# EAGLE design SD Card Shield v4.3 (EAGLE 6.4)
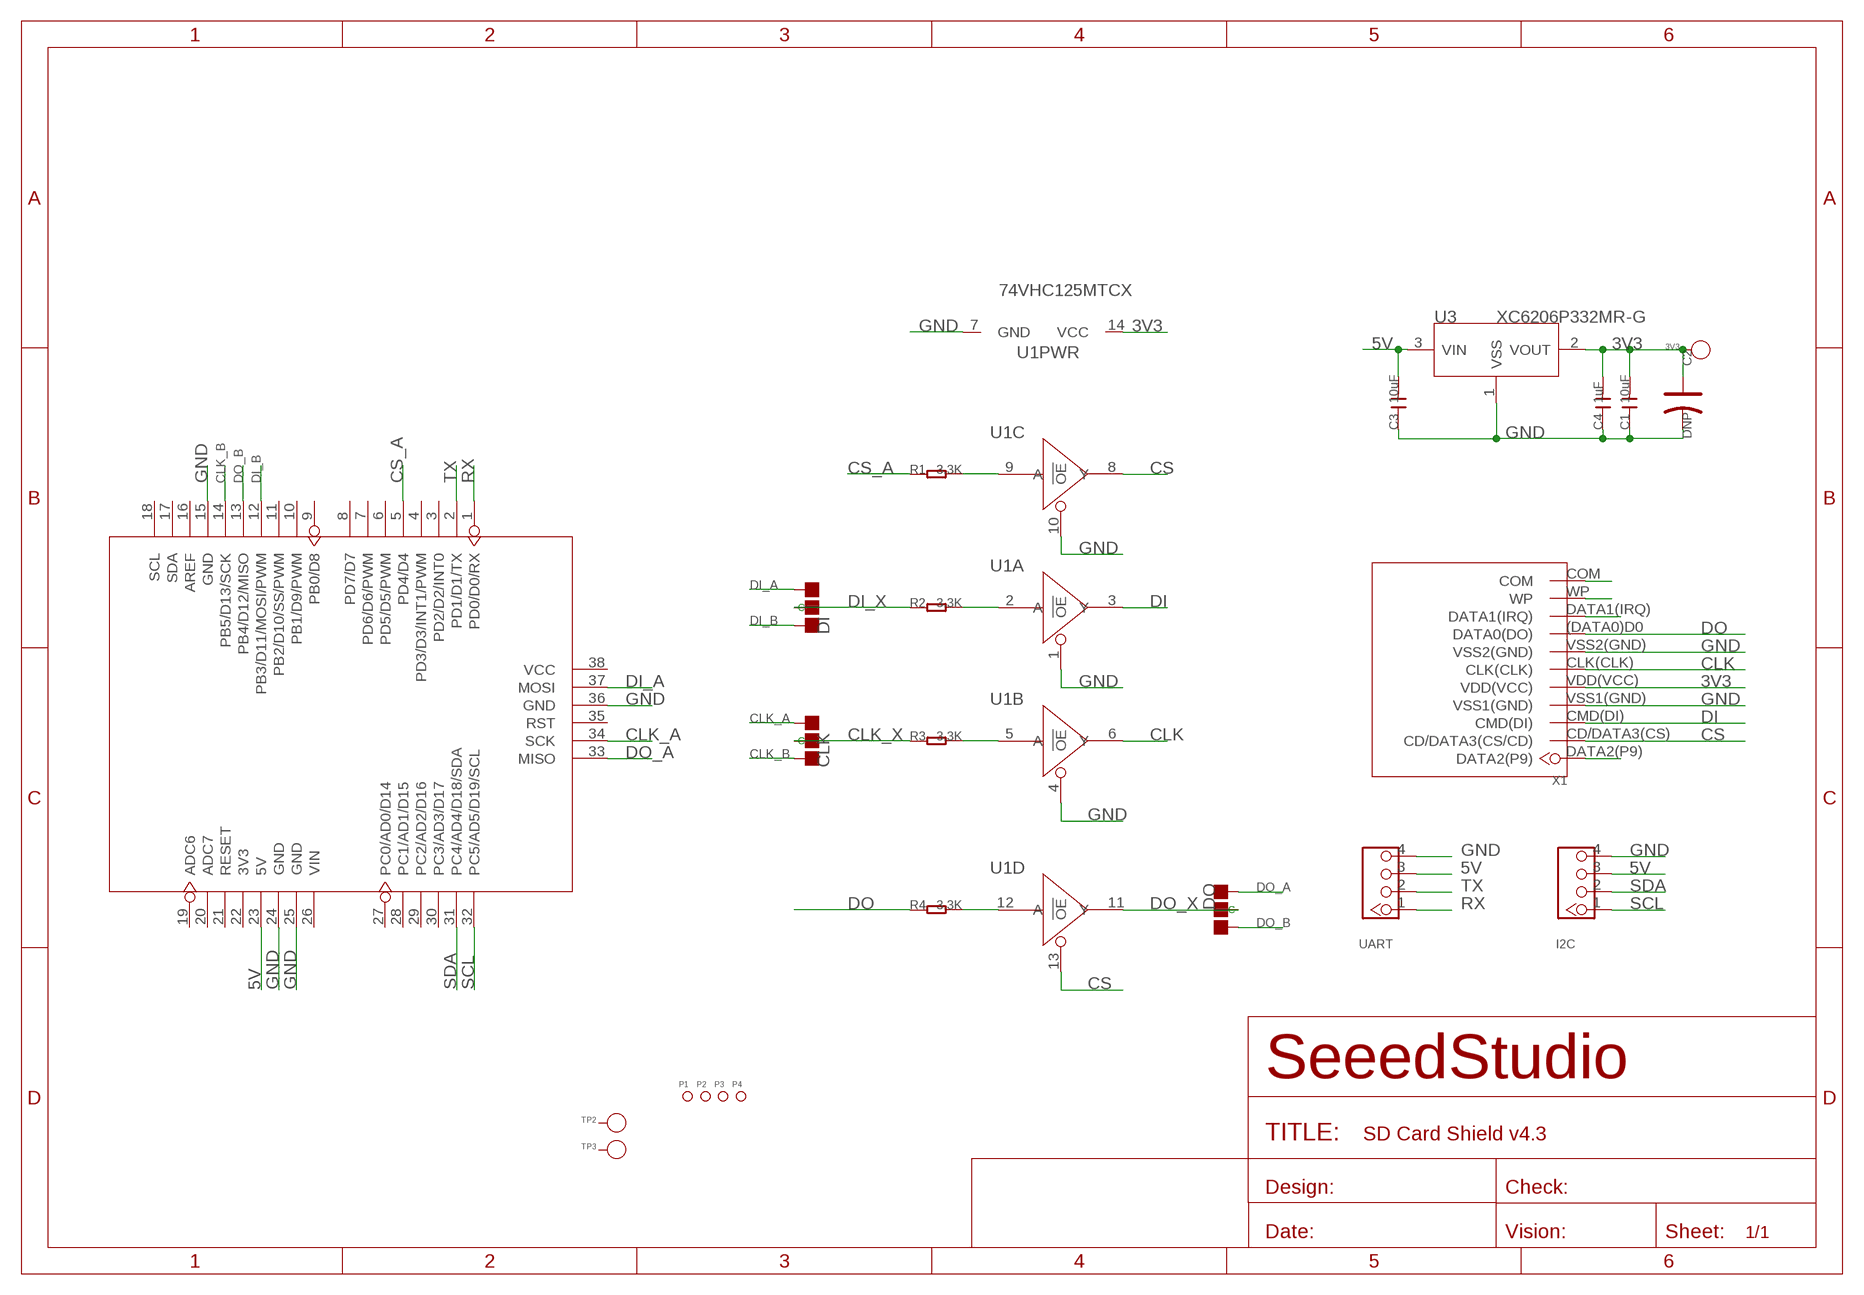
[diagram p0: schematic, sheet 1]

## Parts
3V3  PAD-TEST-POINT'4545'  [TP_4545]
C1  10uF  C-0805  [C0805]
C2  DNP  CAP-AVX-A  [AVX-A]
C3  10uF  C-0805  [C0805]
C4  1uF  C-0805  [C0805]
CLK  PAD-JUMPER-3P-40*40  [3P-SMD-4.1X1.5]
DI  PAD-JUMPER-3P-40*40  [3P-SMD-4.1X1.5]
DO  PAD-JUMPER-3P-40*40  [3P-SMD-4.1X1.5]
I2C  TWIG-4P-2.0-2.0  [4P-2.0]
P1  PAD-MARK'ANNULAR'  [ROUND-MARK-1.0]
P2  PAD-MARK'ANNULAR'  [ROUND-MARK-1.0]
P3  PAD-MARK'ANNULAR'  [ROUND-MARK-1.0]
P4  PAD-MARK'ANNULAR'  [ROUND-MARK-1.0]
R1  3.3K  R-0603  [R0603]
R2  3.3K  R-0603  [R0603]
R3  3.3K  R-0603  [R0603]
R4  3.3K  R-0603  [R0603]
TP2  PAD-TEST-POINT'4545'  [TP_4545]
TP3  PAD-TEST-POINT'4545'  [TP_4545]
U1  74VHC125MTCX  74VHC125PW  [TSSOP14]
U2  ARDUINO-38P'WITH/-SILK'  [ARDUINO-38P-WITH/-SILK-500519002]
U3  XC6206P332MR-G  XC6206MR  [SOT23]
UART  TWIG-4P-2.0-2.0  [4P-2.0]
X1  SDCARDEXTDEVICE  [SDCARDEXTPACKAGE]

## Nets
3V3: 3V3.T C1.2 C2.+ C4.2 U1.14(PWR:VCC) U3.2(VOUT) X1.VDD(VCC)
5V: C3.2 I2C.3 U2.23(5V) U3.3(VIN) UART.3
CLK: U1.6(B:Y) X1.CLK(CLK)
CLK_A: CLK.00(L) U2.34(SCK)
CLK_B: CLK.11(R) U2.14(PB5/D13/SCK)
CLK_X: CLK.MM(C) R3.1
CS: U1.8(C:Y) U1.13(D:!OE) X1.CD/DATA3(CS)(CD/DATA3(CS/CD))
CS_A: R1.1 U2.5(PD4/D4)
DI: U1.3(A:Y) X1.CMD(DI)
DI_A: DI.00(L) U2.37(MOSI)
DI_B: DI.11(R) U2.12(PB3/D11/MOSI/PWM)
DI_X: DI.MM(C) R2.1
DO: R4.1 X1.(DATA0)D0(DATA0(DO))
DO_A: DO.11(R) U2.33(MISO)
DO_B: DO.00(L) U2.13(PB4/D12/MISO)
DO_X: DO.MM(C) U1.11(D:Y)
GND: C1.1 C2.- C3.1 C4.1 I2C.4 U1.1(A:!OE) U1.4(B:!OE) U1.7(PWR:GND) U1.10(C:!OE) U2.15(GND) U2.24(GND) U2.25(GND) U2.36(GND) U3.1(VSS) UART.4 X1.VSS1(GND) X1.VSS2(GND)
N$2: R4.2 U1.12(D:A)
N$3: R3.2 U1.5(B:A)
N$4: R2.2 U1.2(A:A)
N$5: R1.2 U1.9(C:A)
N$6: X1.COM
N$7: X1.WP
N$8: X1.DATA1(IRQ)
N$9: X1.DATA2(P9)
RX: U2.1(PD0/D0/RX) UART.1
SCL: I2C.1 U2.32(PC5/AD5/D19/SCL)
SDA: I2C.2 U2.31(PC4/AD4/D18/SDA)
TX: U2.2(PD1/D1/TX) UART.2
Unconnected: TP2.T TP3.T U2.3(PD2/D2/INT0) U2.4(PD3/D3/INT1/PWM) U2.6(PD5/D5/PWM) U2.7(PD6/D6/PWM) U2.8(PD7/D7) U2.9(PB0/D8) U2.10(PB1/D9/PWM) U2.11(PB2/D10/SS/PWM) U2.16(AREF) U2.17(SDA) U2.18(SCL) U2.19(ADC6) U2.20(ADC7) U2.21(RESET) U2.22(3V3) U2.26(VIN) U2.27(PC0/AD0/D14) U2.28(PC1/AD1/D15) U2.29(PC2/AD2/D16) U2.30(PC3/AD3/D17) U2.35(RST) U2.38(VCC)

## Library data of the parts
3V3 TP2 TP3 = Discrete:PAD-TEST-POINT; PARTNO: DNP
C1 C3 C4 = Discrete:C*: Ceramic Capacitors
C2 = Discrete:CAP*: Electrolytic Capacitors,Tantalum Capacitors and Super Capacitors
CLK DI DO = Discrete:PAD-JUMPER-3P; PARTNO: DNP
I2C UART = Connector:TWIG-4P-2.0
P1-P4 = Discrete:PAD-MARK; PARTNO: DNP
R1-R4 = Discrete:R*
U1 = IC:74V*125: Quad Buffer/Line Driver;3-state
U2 = moudle:ARDUINO-38P
U3 = IC:XC6206: LOW ESR Cap.Compatible Positive Voltage Regulators
X1 = SD card breakout:SDCARDEXTDEVICE

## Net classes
0 default: clearance 0.152 mm

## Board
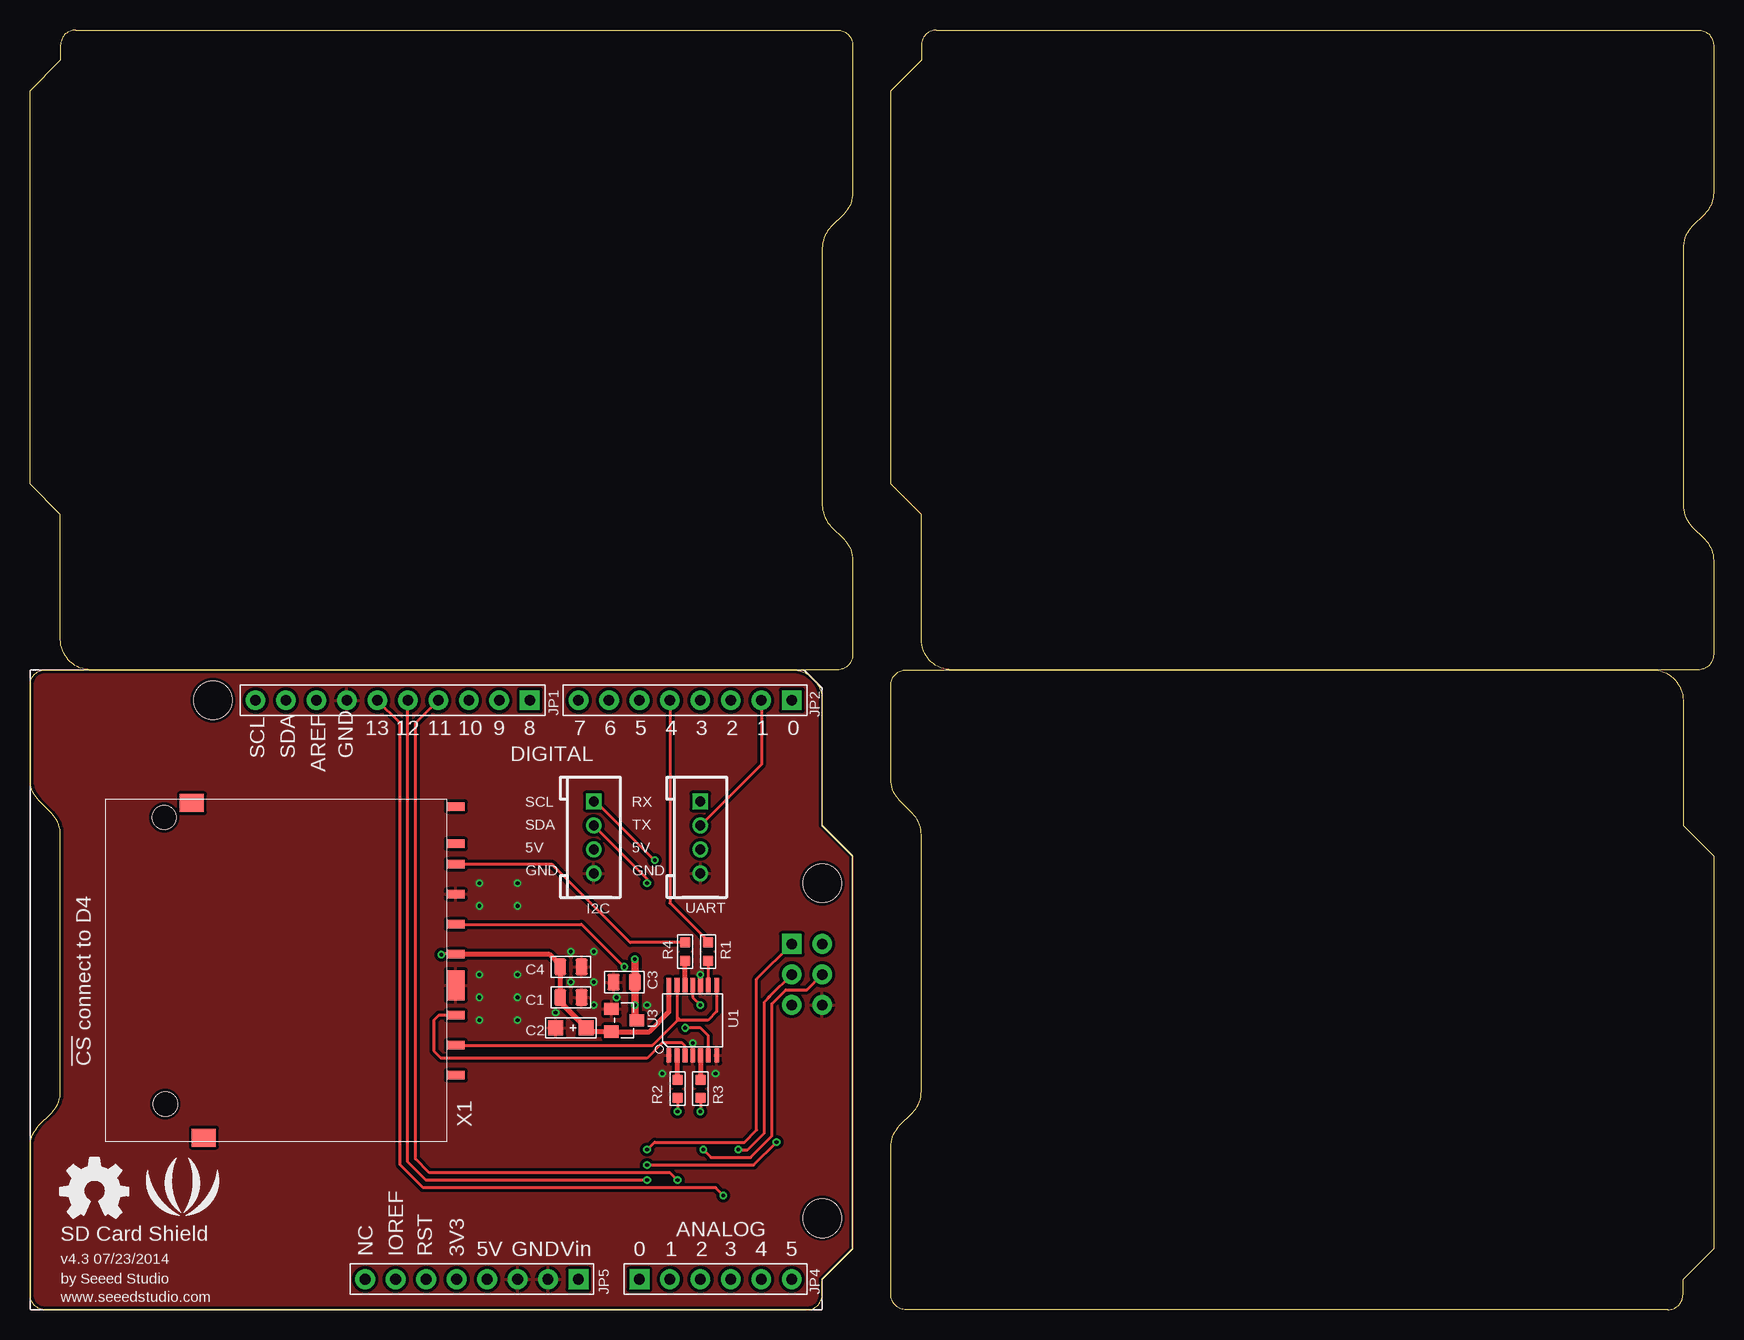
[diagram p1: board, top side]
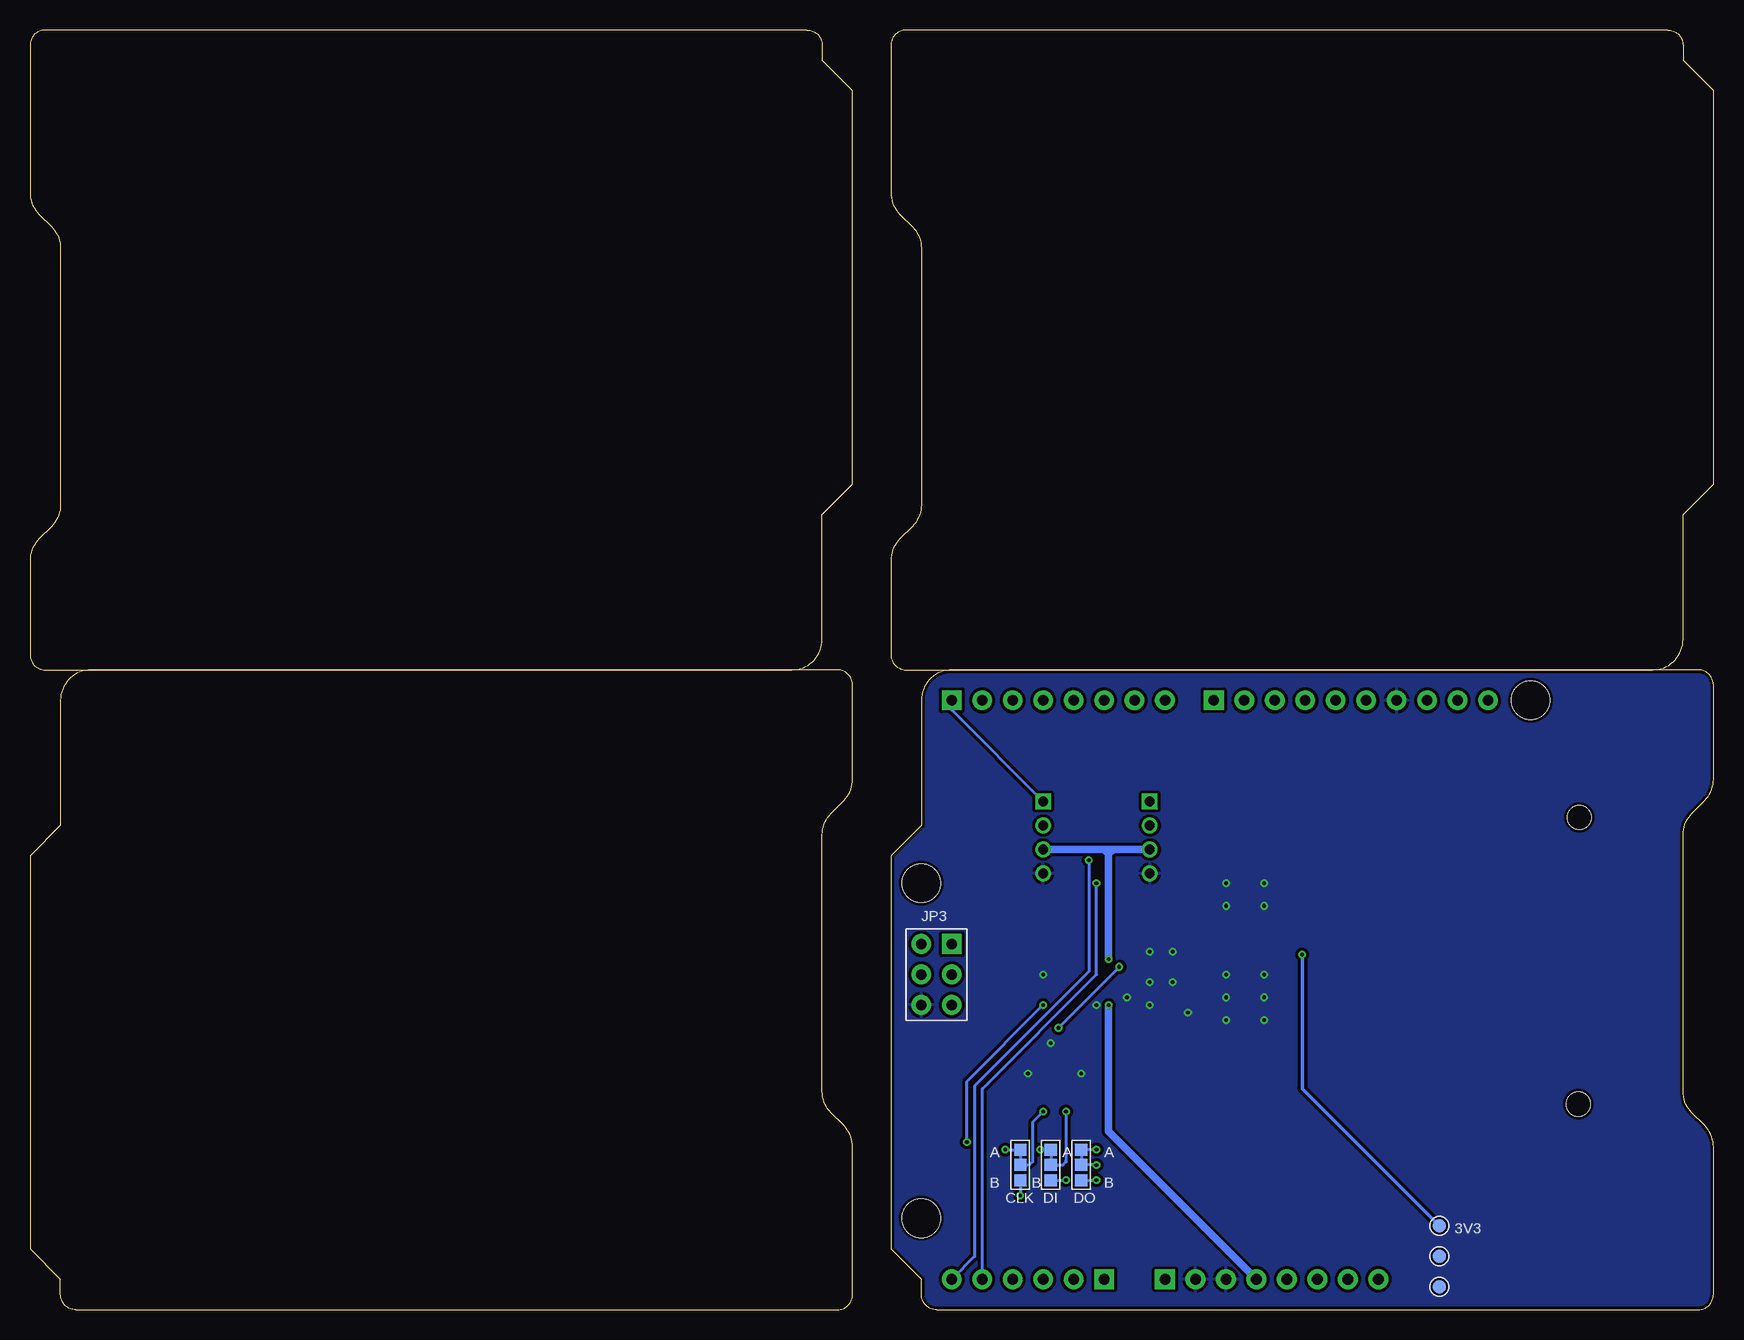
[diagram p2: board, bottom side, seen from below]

Size 140.34 x 106.68 mm. Coordinates in mm from the lower left corner, seen from the top.
Outline: 80 segments
Copper layers (1*16): Top 0.035mm / dielectric 1.5mm / Bottom 0.035mm
Design rules "default *": minimum track width 6mil, minimum drill 12mil, track to track 6mil, track to pad 6mil, pad to pad 6mil, via to via 6mil, smd to smd 0mil, copper to edge 10mil, drill to drill 10mil, minimum pad ring 10mil, minimum via ring 6mil, stop-mask expansion 2mil, vias tented up to drill 100mil, thermal gap 10mil
Holes 2.03 mm at 7.62,111.12 132.72,111.12 132.72,-4.45 7.62,-4.45
tKeepout: area 52.7,26.8 to 59.1,31.9

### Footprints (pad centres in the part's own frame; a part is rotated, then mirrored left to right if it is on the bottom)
TP_4545 = smd 1.143 x 1.143: T 0,0
C0805 = smd 1.016 x 1.397: 1 -0.889,0; 2 0.889,0
AVX-A = smd 1.27 x 1.27: + -1.27,0; - 1.27,0
3P-SMD-4.1X1.5 = smd 1.016 x 1.016: 00 -1.27,0; 11 1.27,0; MM 0,0
4P-2.0 = drill 0.8 pad 1.27 square: 1 -3,0 | drill 0.8 pad 1.27: 2 -1,0; 3 1,0; 4 3,0
ROUND-MARK-1.0 = smd 1.016 x 1.016: P$1 0,0
R0603 = smd 0.889 x 0.889: 1 -0.762,0; 2 0.762,0
TSSOP14 = smd 0.4 x 1.2: 1 -2,-2.925; 2 -1.3,-2.925; 3 -0.65,-2.925; 4 0,-2.925; 5 0.65,-2.925; 6 1.3,-2.925; 7 2,-2.925; 8 2,2.925; 9 1.3,2.925; 10 0.65,2.925; 11 0,2.925; 12 -0.65,2.925; 13 -1.3,2.925; 14 -2,2.925
ARDUINO-38P-WITH/-SILK-500519002 = drill 0.889 pad 1.651 square: 1 63.5,50.8; 9 41.656,50.8; 26 45.72,2.54; 27 50.8,2.54; 33 63.5,30.48 | drill 0.889 pad 1.651: 2 60.96,50.8; 3 58.42,50.8; 4 55.88,50.8; 5 53.34,50.8; 6 50.8,50.8; 7 48.26,50.8; 8 45.72,50.8; 10 39.116,50.8; 11 36.576,50.8; 12 34.036,50.8; 13 31.496,50.8; 14 28.956,50.8; 15 26.416,50.8; 16 23.876,50.8; 17 21.336,50.8; 18 18.796,50.8; 19 27.94,2.54; 20 30.48,2.54; 21 33.02,2.54; 22 35.56,2.54; 23 38.1,2.54; 24 40.64,2.54; 25 43.18,2.54; 28 53.34,2.54; 29 55.88,2.54; 30 58.42,2.54; 31 60.96,2.54; 32 63.5,2.54; 34 63.5,27.94; 35 63.5,25.4; 36 66.04,25.4; 37 66.04,27.94; 38 66.04,30.48 | hole 3.2: 15.24,50.8; 66.04,35.56; 66.04,7.62
SOT23 = smd 1.016 x 1.2: 1 -0.95,-1.06; 2 0.95,-1.06; 3 0,1.06
SDCARDEXTPACKAGE = smd 1.5 x 0.7: (DATA0)D0 -15.8,-9.2; CD/DATA3(CS) -15.8,5.9; CLK(CLK) -15.8,-4.2; CMD(DI) -15.8,3.4; DATA1(IRQ) -15.8,-10.9; DATA2(P9) -15.8,8.4; VDD(VCC) -15.8,-1.7; VSS2(GND) -15.8,-6.7; WP -15.8,-14 | smd 2 x 1.5: COM 6.2,-14.3; P$2 5.2,13.6 | smd 1.5 x 2.5: VSS1(GND) -15.8,0.9 | hole 2: 8.4,10.8; 8.5,-13.1

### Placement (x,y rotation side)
3V3  22.86,6.99 0 bottom
C1  45.09,26.04 180 top
C2  45.09,23.5 180 top
C3  49.53,27.3 0 top
C4  45.09,28.57 180 top
CLK  57.78,12.06 270 bottom
DI  55.24,12.06 270 bottom
DO  52.7,12.06 90 bottom
I2C  46.99,39.37 270 top
P1  not placed on the board
P2  not placed on the board
P3  not placed on the board
P4  not placed on the board
R1  56.52,29.84 270 top
R2  53.98,18.41 90 top
R3  55.88,18.41 90 top
R4  54.61,29.84 270 top
TP2  22.86,4.45 0 bottom
TP3  22.86,1.91 0 bottom
U1  55.24,24.13 0 top
U2  0,0 0 top
U3  49.53,24.13 270 top
U$1  [OSHW_FILLX200_NOTEXT]  2.54,7.62 0 top
U$2  [LOGO_SILK]  12.7,9.53 0 top
UART  55.88,39.37 270 top
X1  19.68,27.94 180 top

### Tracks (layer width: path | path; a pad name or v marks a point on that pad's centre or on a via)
3V3  (via drill 0.3 pad 0.64)
  Top 0.254: X1.VDD(VCC) 34.34,29.64 v34.29,29.59
  Top 0.406: X1.VDD(VCC) 43.26,29.64 44.32,28.57 C4.2 C1.2 44.2,25.65 C2.+ 46.04,23.18 U3.2 51.63,23.18 53.24,24.8 U1.14
  Bottom 0.305: v34.29,29.59 34.29,18.41 3V3.T
5V  (via drill 0.3 pad 0.64)
  Top 0.406: 50.67,27.05 C3.2
  Top 0.61: U3.3 50.42,24.3 v50.42,25.4 C3.2 v50.42,29.21
  Bottom 0.61: UART.3 50.42,38.37 | 50.42,38.37 I2C.3 | v50.42,29.21 50.42,37.97 | 50.42,37.97 50.42,38.37 | v50.42,25.4 50.42,14.86 U2.23 | 50.42,37.97 50.04,38.35 | 50.42,37.97 50.8,38.35
CLK  (via drill 0.3 pad 0.64)
  Top 0.254: 35.49,32.13 45.97,32.13 v49.53,28.57 | U1.6 56.55,22.83 55.88,23.5 v54.61,23.5
  Top 0.406: 35.49,32.13 X1.CLK(CLK)
  Bottom 0.254: v54.61,23.5 v49.53,28.57
CLK_A  (via drill 0.3 pad 0.64)
  Top 0.254: U2.34 61.66,26.1 61.47,25.91 61.21,25.65 61.21,14.73 59.82,13.34 v59.05,13.34
  Bottom 0.254: v59.05,13.34 CLK.00 57.78,12.06
CLK_B  (via drill 0.3 pad 0.64)
  Top 0.254: v57.78,9.53 57.15,10.16 32.77,10.16 30.86,12.06 30.86,48.9 U2.14
  Bottom 0.254: CLK.11 v57.78,9.53
CLK_X  (via drill 0.3 pad 0.64)
  Top 0.254: R3.1 v55.88,16.51
  Bottom 0.254: v55.88,16.51 56.77,15.62 56.77,12.32 57.02,12.06 CLK.MM
CS
  Top 0.254: X1.CD/DATA3(CS) 51.88,22.04 53.98,24.13 | U1.8 57.24,24.86 56.52,24.13 54.23,24.13 | 54.23,24.13 53.98,24.13 | U1.13 53.95,24.16 53.98,24.13 | 54.23,24.13 53.98,24.38
CS_A
  Top 0.254: U2.5 53.34,33.91 56.01,31.24 56.13,31.11 56.52,30.73 R1.1
DI
  Top 0.254: X1.CMD(DI) 34.06,24.54 33.66,24.13 33.66,21.59 34.29,20.95 51.44,20.95 52.7,22.23 54.36,22.23 54.59,21.99 U1.3
DI_A  (via drill 0.3 pad 0.64)
  Top 0.254: U2.37 64.77,26.67 63.02,26.67 61.85,25.5 61.85,14.48 60.07,12.7 56.77,12.7 v56.13,13.34
  Bottom 0.254: v56.13,13.34 DI.00 55.24,12.06
DI_B  (via drill 0.3 pad 0.64)
  Top 0.254: v53.98,10.79 53.34,11.43 33.27,11.43 32.13,12.57 32.13,48.9 U2.12
  Bottom 0.254: DI.11 v53.98,10.79
DI_X  (via drill 0.3 pad 0.64)
  Top 0.254: R2.1 v53.98,16.51
  Bottom 0.254: v53.98,16.51 53.98,12.57 53.98,12.45 53.98,12.32 54.23,12.06 DI.MM
DO
  Top 0.254: R4.1 50.04,30.61 44.32,36.32 43.81,36.83 43.51,37.14 X1.(DATA0)D0
DO_A  (via drill 0.3 pad 0.64)
  Top 0.254: v51.44,13.34 52.07,13.97 59.56,13.97 60.58,14.99 60.58,27.56 U2.33
  Bottom 0.254: v51.44,13.34 DO.11 52.7,12.06
DO_B  (via drill 0.3 pad 0.64)
  Top 0.254: v51.44,10.79 33.02,10.79 31.5,12.32 U2.13
  Bottom 0.254: DO.00 v51.44,10.79
DO_X  (via drill 0.3 pad 0.64)
  Top 0.254: v51.44,12.06 60.33,12.06 v62.23,13.97 | U1.11 55.24,26.04 v55.88,25.4
  Bottom 0.254: v51.44,12.06 DO.MM | v55.88,25.4 62.23,19.05 v62.23,13.97
GND  (via drill 0.3 pad 0.64)
  other vias: 55.24,22.23 46.99,27.3 46.99,25.4 48.9,26.04 46.99,29.84 45.09,27.3 40.64,24.13 43.81,24.77 45.09,29.84 51.44,25.4 57.15,19.68 52.7,19.68 55.88,27.94 37.47,27.94 40.64,27.94 40.64,26.04 37.47,26.04 37.47,35.56 40.64,35.56 40.64,33.66 37.47,33.66 37.47,24.13
  pour Bottom (isolate 0.254): 0,53.34 68.58,53.34 68.58,0 0,0
  pour Top (isolate 0.254): 0,53.34 68.58,53.34 68.58,0 0,0
N$2
  Top 0.406: U1.12 54.59,29.07 R4.2
N$3
  Top 0.406: U1.5 55.9,19.19 R3.2
N$4
  Top 0.406: U1.2 53.95,19.21 R2.2
N$5
  Top 0.254: U1.9 56.55,29.18 56.52,29.21 R1.2
  Top 0.406: 56.55,29.05 R1.2
RX
  Bottom 0.254: U2.1 63.5,49.99 UART.1
SCL  (via drill 0.3 pad 0.64)
  Top 0.254: I2C.1 47.16,42.37 v52.07,37.47
  Bottom 0.254: v52.07,37.47 52.07,28.19 61.59,18.67 61.59,4.45 U2.32
SDA  (via drill 0.3 pad 0.64)
  Top 0.254: v51.44,35.56 51.44,35.92 I2C.2
  Bottom 0.254: U2.31 60.96,18.41 51.44,27.94 v51.44,35.56
TX
  Top 0.254: U2.2 60.96,45.45 UART.2

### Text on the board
tPlace: DIGITAL | SCL | RX | SDA | TX | 5V | 5V | GND | GND | !CS! connect to D4 | SD Card Shield | v4.3 07/23/2014 | by Seeed Studio | www.seeedstudio.com
bPlace: A | A | A | B | B | B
